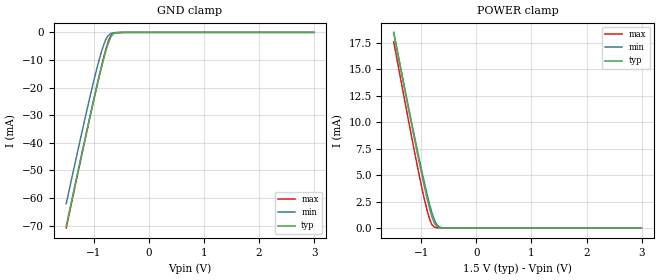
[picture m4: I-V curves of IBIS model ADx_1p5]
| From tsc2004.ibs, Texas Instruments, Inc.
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| Model 1.5 V ADx
[Model]   ADx_1p5
Model_type  Input
Vinl = 0.3
Vinh = 1.05
|   typ   min   max
|   (nom PVT)   (Fast PVT)   (slow PVT)
C_comp   7.01584E-12   6.71223E-12   7.51761E-12
| Where   nom PVT is  Nominal Process, 3.3V, 25C
|   Fast PVT is Strong Process, 3.6V, -40C
|   Slow PVT is Weak Process, 3.0V, 85C
|C_comp - from L-C Tank method, L = 1nH, peak frequency ~ 1.9GHz
[Model Spec]   | power 1.5, 1.2, 1.8 V
Vinl   0.3   0.24   0.54
Vinh   1.05   0.84   1.26
[Voltage Range]   1.5   1.2   1.8
[Temperature Range]   30   88   -40
|Ambient Temperature Range 27   85   -40
[Power Clamp Reference]   1.5   1.2   1.8
[GND Clamp Reference]   0   0   0
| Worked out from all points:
|   GND clamp passes 1 mA (typ) near -0.67 V on its own axis
|   POWER clamp passes 1 mA (typ) near -0.80 V on its own axis
[GND Clamp]
|   Voltage   I(typ)   I(min)   I(max)
-1.5V     -70.22mA   -62.07mA   -70.87mA
-1.142V   -37.09mA   -29.72mA   -37.4mA
-985mV    -23.07mA   -16.37mA   -23.15mA
-899.3mV  -15.81mA   -9.735mA   -15.68mA
-837.6mV  -10.86mA   -5.578mA   -10.53mA
-783.4mV  -6.895mA   -2.724mA   -6.373mA
-723.3mV  -3.213mA   -917.5uA   -2.553mA
-703.2mV  -2.276mA   -574.5uA   -1.648mA
-663.9mV  -968.6uA   -258.3uA   -600.6uA
-614.2mV  -264.6uA   -96.64uA   -224.2uA
-459.5mV  -5.672uA   -7.74uA    -26.44uA
2.995V    0A         0A         0A
[POWER Clamp]
|   Voltage   I(typ)   I(min)   I(max)
-1.5V     18.46mA    18.45mA    17.57mA
-1.162V   9.417mA    9.639mA    8.251mA
-1.024V   5.897mA    6.219mA    4.663mA
-948.7mV  4.053mA    4.424mA    2.845mA
-861.7mV  2.107mA    2.515mA    1.079mA
-817.6mV  1.279mA    1.662mA    450.8uA
-798.1mV  960.6uA    1.332mA    274.4uA
-760mV    474.8uA    772.6uA    102.1uA
-715.3mV  164uA      341.6uA    32.47uA
-655.2mV  32.89uA    86.09uA    16.48uA
-510.6mV  1.333uA    1.582uA    1.305uA
2.995V    0A         0A         0A
